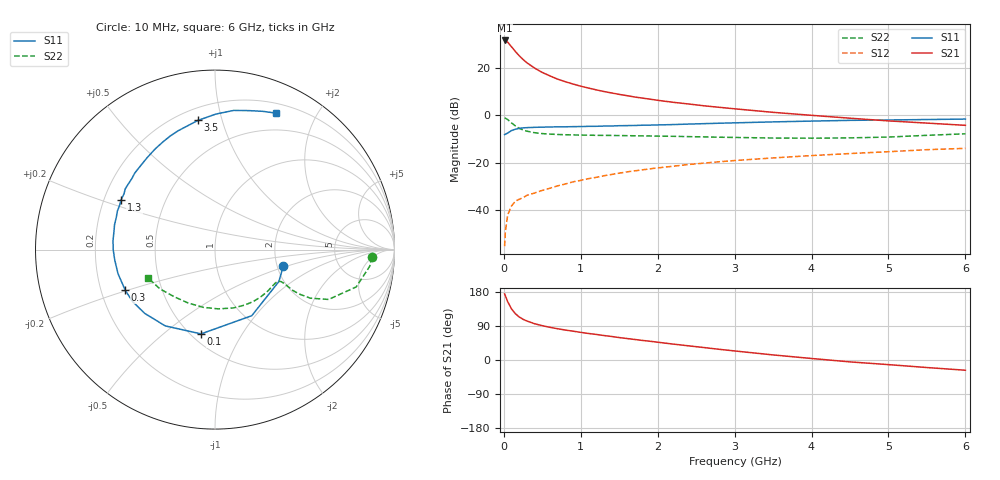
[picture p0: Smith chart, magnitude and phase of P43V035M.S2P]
! SIEMENS Small Signal Semiconductors
! BFP182
! Si NPN RF Bipolar Junction Transistor in SOT143
! VCE = 3 V  IC = 35 mA
! Common Emitter S-Parameters:  March  1996
# GHz  S  MA  R  50
!  f  S11  S21  S12  S22
! GHz  MAG  ANG  MAG  ANG  MAG  ANG  MAG  ANG
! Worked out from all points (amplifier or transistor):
!   36 points, 10 MHz to 6 GHz, reference 50 ohm
!   highest |S21| = 31.7 dB at 10 MHz (marker M1)
!   |S21| within 3 dB of that: start of sweep to 108.2 MHz
!   unconditionally stable (mu >= 1): start of sweep to 15.82 MHz; 330.4 MHz to end of sweep
!   at 250 MHz: K = 0.88, MSG = 29.2 dB, |S12| = -34.8 dB
!   at 1.4 GHz: K = 1.53, MAG = 13.0 dB, |S12| = -25.0 dB
!   at 6 GHz: K = 1.06, MAG = 3.4 dB, |S12| = -14.0 dB
!   S11 on the Smith chart (normalised r, x): 10 MHz: 2.16, -0.46; 100 MHz: 0.56, -0.68; 300 MHz: 0.30, -0.20; 1.3 GHz: 0.27, +0.23; 3.5 GHz: 0.28, +0.84; 6 GHz: 0.30, +1.50
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0.01  0.3916 -13.3  38.44 174.4  0.0017 78.5  0.8745 -2.7
0.02  0.3978 -26.6  38.2 169.3  0.0035 76.5  0.8675 -6.1
0.05  0.4214 -60.9  35.33 153.9  0.0078 72.7  0.8139 -14.8
0.1  0.476 -99.4  28.27 134.8  0.0121 55.6  0.6909 -23.7
0.15  0.5075 -123.1  22.43 122.1  0.0152 50.8  0.5961 -27.0
0.2  0.5286 -137.7  18.25 113.5  0.0167 49.1  0.5312 -27.8
0.25  0.5429 -147.8  15.2 107.4  0.0181 49.1  0.4899 -27.7
0.3  0.5489 -155.6  12.97 102.9  0.0203 50.0  0.4619 -27.0
0.4  0.5569 -166.1  9.989 95.7  0.0227 52.4  0.4284 -26.1
0.5  0.5617 -174.2  8.074 90.5  0.0258 53.1  0.4104 -25.8
0.6  0.5671 -179.9  6.822 86.2  0.0287 56.0  0.4003 -26.2
0.7  0.5705 174.8  5.817 82.5  0.0322 57.2  0.3935 -26.9
0.8  0.5718 169.9  5.141 79.0  0.0352 58.3  0.3882 -27.8
1.1  0.5846 158.6  3.78 70.0  0.0457 59.3  0.38 -31.9
1.3  0.5921 152.1  3.194 64.6  0.0526 58.7  0.3762 -35.2
1.7  0.6099 139.1  2.442 54.2  0.0668 57.4  0.3691 -42.7
2.2  0.6374 126.1  1.889 42.0  0.0838 54.0  0.3597 -53.2
2.8  0.6806 111.4  1.479 28.2  0.104 48.8  0.3439 -67.6
3.5  0.7262 97.5  1.157 13.4  0.1254 42.4  0.3306 -87.0
4.5  0.7826 82.3  0.869 -5.0  0.1553 33.2  0.3331 -116.8
5.5  0.8148 71.0  0.685 -19.9  0.1875 24.2  0.3774 -144.7
6  0.8333 65.8  0.614 -27.0  0.2001 18.6  0.4063 -157.5
